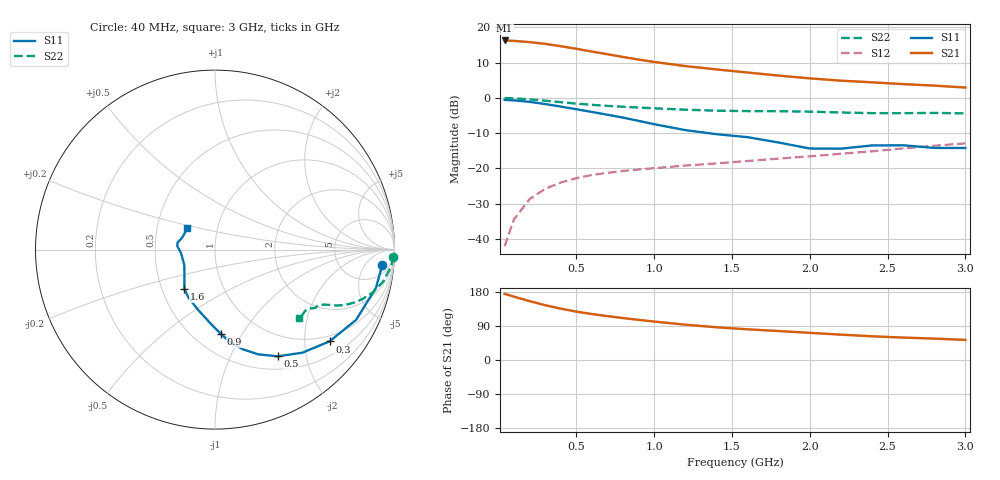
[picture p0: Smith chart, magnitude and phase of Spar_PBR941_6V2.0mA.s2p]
! Filename:  PBR941L.S2P  Version:  3.0
! NXP part #:  PBR941  Date: July 1998
! Bias condition:  Vce=6V, Ic=2.0mA
#  MHz  S  MA  R 50
! Freq  S11  S21  S12  S22
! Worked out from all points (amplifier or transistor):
!   21 points, 40 MHz to 3 GHz, reference 50 ohm
!   highest |S21| = 16.3 dB at 40 MHz (marker M1)
!   |S21| within 3 dB of that: start of sweep to 581.9 MHz
!   unconditionally stable (mu >= 1): 1.754 GHz to end of sweep
!   at 300 MHz: K = 0.26, MSG = 20.6 dB, |S12| = -25.8 dB
!   at 1 GHz: K = 0.74, MSG = 15.1 dB, |S12| = -20.0 dB
!   at 3 GHz: K = 1.02, MAG = 7.1 dB, |S12| = -12.9 dB
!   lowest NFmin = 1.04 dB at 500 MHz
!   S11 on the Smith chart (normalised r, x): 40 MHz: 10, -14; 300 MHz: 0.84, -2.61; 500 MHz: 0.68, -1.53; 900 MHz: 0.67, -0.81; 1.6 GHz: 0.65, -0.31; 3 GHz: 0.72, +0.18
40  0.9356 -5.4  6.528 174.7  0.007862 86.6  0.9945 -2.3
100  0.9217 -13.4  6.432 167.2  0.01883 81.5  0.985 -5.6
200  0.8784 -26.4  6.182 155.4  0.03655 75.2  0.9537 -10.8
300  0.8179 -38.7  5.846 144.7  0.0511 70.0  0.9122 -15.1
400  0.753 -49.7  5.412 135.5  0.0628 65.4  0.8687 -18.4
500  0.6899 -59.5  4.977 127.7  0.07236 62.4  0.8295 -20.9
600  0.6317 -67.5  4.546 121.4  0.08048 60.5  0.7962 -22.6
700  0.5767 -74.4  4.163 115.8  0.08615 59.5  0.7697 -23.8
800  0.5252 -80.5  3.809 110.7  0.09168 59.1  0.7486 -24.6
900  0.4719 -85.9  3.496 105.9  0.09621 58.9  0.729 -25.2
1000  0.4234 -91.9  3.235 101.5  0.1005 59.0  0.7111 -25.7
1200  0.349 -105.6  2.827 93.2  0.1095 60.1  0.6797 -26.8
1400  0.3054 -119.1  2.535 86.4  0.1175 61.5  0.6577 -28.2
1600  0.2769 -128.0  2.29 81.0  0.1272 64.1  0.6494 -29.3
1800  0.2326 -137.0  2.071 76.4  0.1375 66.9  0.6469 -30.1
2000  0.1913 -153.5  1.891 71.7  0.148 68.8  0.6378 -30.8
2200  0.1902 -174.1  1.754 66.9  0.1609 70.5  0.62 -32.0
2400  0.2114 174.6  1.662 62.5  0.1745 72.2  0.6074 -34.1
2600  0.2125 169.4  1.567 59.2  0.1917 74.1  0.6072 -36.7
2800  0.1946 160.2  1.492 56.5  0.2094 75.3  0.6113 -38.4
3000  0.1946 142.2  1.402 53.0  0.2262 75.8  0.6033 -39.4
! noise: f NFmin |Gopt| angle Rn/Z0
500  1.038  0.588  13.28  0.379
900  1.111  0.497  29.36  0.372
1000  1.168  0.448  32.72  1.369
2000  1.951  0.206  103.6  0.22
